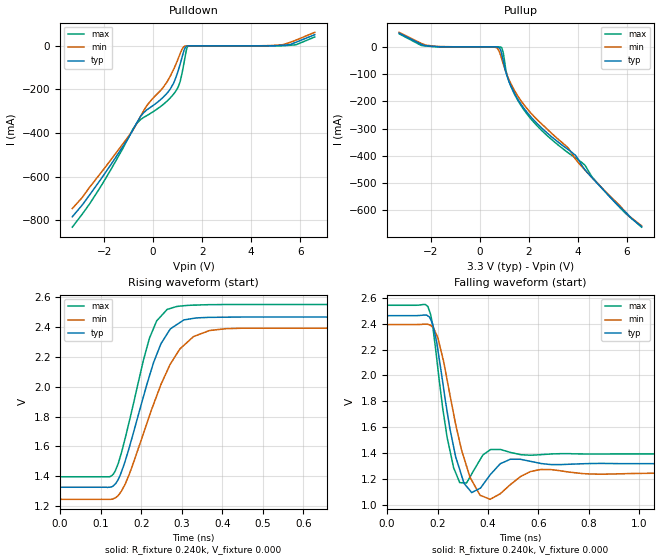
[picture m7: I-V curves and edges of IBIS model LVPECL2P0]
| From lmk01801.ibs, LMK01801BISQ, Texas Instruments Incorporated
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|   Model LVPECL2P0V
[Model]   LVPECL2P0
Model_type   Output
Polarity   Non-Inverting
Vmeas = 1.99
Vref = 0
Cref = .3pF
Rref = 240
|   typ   min   max
|   (nom PVT)   (fast PVT)   (slow PVT)
C_comp   0.2109p   0.1807p   0.2310p
|C_comp (Low state)   0.2109p   0.1807p   0.2310p
|C_comp (High state)   0.9933p   0.9197p   1.0724p
[Voltage Range]   3.3   3.135   3.465
[Temperature Range]   45   125   -40
[Pullup Reference]   3.3   3.135   3.465
[Pulldown Reference]   0   0   0
[Power Clamp Reference]   3.3   3.135   3.465
[GND Clamp Reference]   0   0   0
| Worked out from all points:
|   slope of the pulldown table from 0 to 0.495 V, typ, clamps not added: 10.4 ohm
|   falling waveform, R_fixture 0.240k, V_fixture 0.000: 20-80 % time 55ps typ, 72.1ps min, 44.7ps max; typ from 2.46 V to 1.32 V
|   rising waveform, R_fixture 0.240k, V_fixture 0.000: 20-80 % time 75.1ps typ, 95.6ps min, 61.9ps max; typ from 1.33 V to 2.47 V
[Pulldown]
|   Voltage   I(typ)   I(min)   I(max)
-3.3V     -785mA     -747.1mA   -832.6mA
-2.166V   -617.6mA   -588.2mA   -651.2mA
-686.4mV  -357.3mA   -360mA     -358.4mA
-255.7mV  -293.6mA   -274.3mA   -320.1mA
575.8mV   -216.4mA   -163.5mA   -252.9mA
932.3mV   -143.9mA   -83.44mA   -206.3mA
1.096V    -86.76mA   -37.35mA   -166.4mA
1.304V    -8.601mA   -1.187mA   -50.55mA
1.422V    -244.7uA   -92.18uA   -1.848mA
5.244V    2.364mA    5.07mA     347.1uA
5.838V    16.95mA    26.83mA    5.377mA
6.595V    51.39mA    62.18mA    40.83mA
[Pullup]
|   Voltage   I(typ)   I(min)   I(max)
-3.3V     50.87mA    53.61mA    48.19mA
-2.206V   4.569mA    6.157mA    3.254mA
561mV     -1.357uA   -107.4uA   -21.23nA
709.5mV   -258.2uA   -4.509mA   -735.3nA
877.8mV   -22.94mA   -41.64mA   -2.132mA
1.071V    -97.72mA   -95.94mA   -91.62mA
1.254V    -142.6mA   -134.3mA   -143.5mA
1.947V    -243.6mA   -229.8mA   -250.1mA
3.887V    -398mA     -411.4mA   -408mA
4.283V    -451.8mA   -452.5mA   -435mA
5.313V    -552.1mA   -549mA     -552.7mA
6.595V    -660mA     -657.5mA   -662.5mA
[Ramp]
R_load = 240
|   typ   min   max
dV/dt_r   0.662924/7.51377e-11   0.65498/9.56481e-11   0.6703/6.18644e-11
dV/dt_f   0.68438/5.49359e-11   0.681221/7.215e-11   0.687432/4.47236e-11
[Falling Waveform]
R_fixture = 0.240k
V_fixture = 0.000
V_fixture_min = 0.000
V_fixture_max = 0.000
C_fixture = 0.000
|  time   V(typ)   V(min)   V(max)
0s        2.461V     2.392V     2.541V
161.7ps   2.459V     2.394V     2.532V
196.7ps   2.257V     2.312V     2.135V
237.9ps   1.724V     1.967V     1.524V
287.9ps   1.275V     1.487V     1.174V
335.5ps   1.097V     1.192V     1.24V
408.8ps   1.235V     1.045V     1.427V
488.4ps   1.354V     1.158V     1.407V
608.4ps   1.322V     1.275V     1.389V
1.999ns   1.32V      1.245V     1.395V
[Rising Waveform]
R_fixture = 0.240k
V_fixture = 0.000
V_fixture_min = 0.000
V_fixture_max = 0.000
C_fixture = 0.000
|  time   V(typ)   V(min)   V(max)
0s        1.326V     1.245V     1.396V
132ps     1.338V     1.25V      1.417V
143.5ps   1.38V      1.272V     1.488V
160.2ps   1.5V       1.346V     1.653V
220ps     2.071V     1.804V     2.324V
248.7ps   2.289V     2.016V     2.473V
287.9ps   2.417V     2.222V     2.538V
328.8ps   2.458V     2.336V     2.547V
408.8ps   2.466V     2.389V     2.551V
1.999ns   2.466V     2.392V     2.551V
